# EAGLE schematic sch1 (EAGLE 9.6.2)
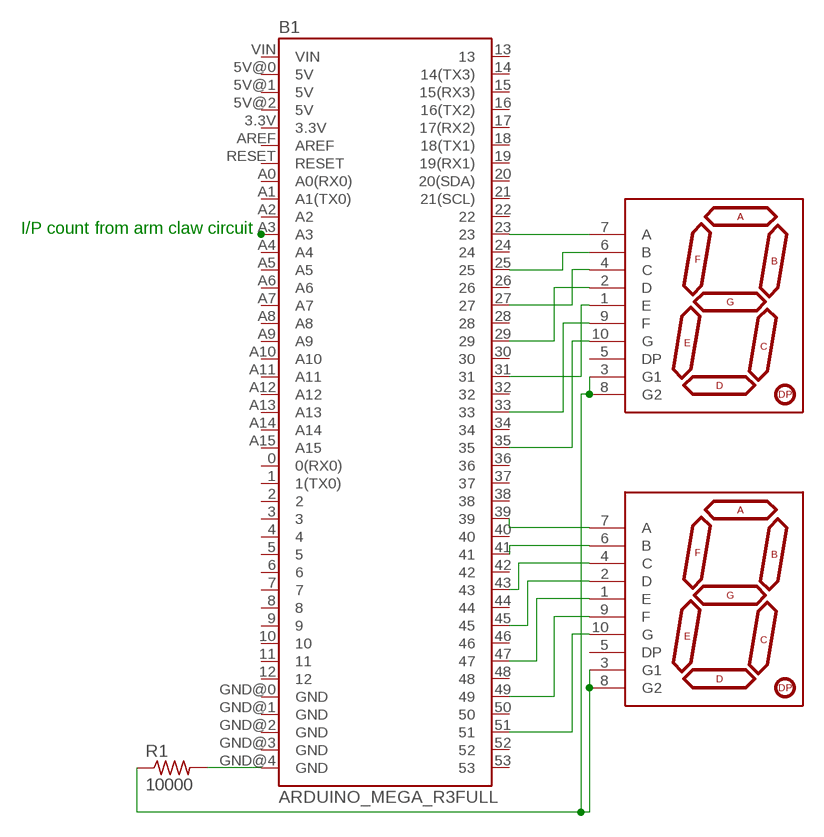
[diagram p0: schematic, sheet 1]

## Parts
B1  ARDUINO_MEGA_R3FULL  [ARDUINO_MEGA]
R1  10000  R-US_0309/12  [0309/12]
U$1  YSD-1601AR4B-8  7-SEGMENT-1DIGIT-1INCH-RED  [7-SEGMENT-1"PTH]
U$2  YSD-1601AR4B-8  7-SEGMENT-1DIGIT-1INCH-RED  [7-SEGMENT-1"PTH]

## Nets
N$1: B1.23 U$1.7(A)
N$2: B1.25 U$1.6(B)
N$3: B1.27 U$1.4(C)
N$4: B1.29 U$1.2(D)
N$5: B1.31 U$1.1(E)
N$6: B1.33 U$1.9(F)
N$7: B1.35 U$1.10(G)
N$8: B1.A3
N$9: B1.GND@4(GND) R1.2
N$10: B1.43 U$2.4(C)
N$11: R1.1 U$1.3(G1) U$1.8(G2) U$2.3(G1) U$2.8(G2)
N$12: B1.39 U$2.7(A)
N$13: B1.41 U$2.6(B)
N$14: B1.45 U$2.2(D)
N$15: B1.47 U$2.1(E)
N$16: B1.49 U$2.9(F)
N$17: B1.51 U$2.10(G)
Unconnected: B1.0(0(RX0)) B1.1(1(TX0)) B1.2 B1.3 B1.3.3V B1.4 B1.5 B1.5V@0(5V) B1.5V@1(5V) B1.5V@2(5V) B1.6 B1.7 B1.8 B1.9 B1.10 B1.11 B1.12 B1.13 B1.14(14(TX3)) B1.15(15(RX3)) B1.16(16(TX2)) B1.17(17(RX2)) B1.18(18(TX1)) B1.19(19(RX1)) B1.20(20(SDA)) B1.21(21(SCL)) B1.22 B1.24 B1.26 B1.28 B1.30 B1.32 B1.34 B1.36 B1.37 B1.38 B1.40 B1.42 B1.44 B1.46 B1.48 B1.50 B1.52 B1.53 B1.A0(A0(RX0)) B1.A1(A1(TX0)) B1.A2 B1.A4 B1.A5 B1.A6 B1.A7 B1.A8 B1.A9 B1.A10 B1.A11 B1.A12 B1.A13 B1.A14 B1.A15 B1.AREF B1.GND@0(GND) B1.GND@1(GND) B1.GND@2(GND) B1.GND@3(GND) B1.RESET B1.VIN U$1.5(DP) U$2.5(DP)

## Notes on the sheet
- I/P count from arm claw circuit

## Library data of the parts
B1 = SparkFun-Boards:ARDUINO_MEGA_R3: Arduino Mega R3 ATmega2560 R3 compatible footprint. SparkFun Products: Arduino Mega 2560 R3
R1 = adafruit:R-US_: RESISTOR, American symbol
U$1 U$2 = SparkFun-LED:7-SEGMENT-1DIGIT-1INCH: 7-Segment Display, single digit, 1" EZ is for kits. Pads are only exposed on the bottom side to help prevent soldering in upside down. Datasheet (Red) Datasheet (Blue) SparkFun Products 7-Segment Display - LED (Red) (COM-08546) 7-Segment Display - LED (Blue) (COM-09191); PROD_ID: COMP-08615

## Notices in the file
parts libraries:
SparkFun-Boards: Licensing: Creative Commons ShareAlike 4.0 International - https://creativecommons.org/licenses/by-sa/4.0
